FUNCTION "GeneralConditions" : VOID
TITLE =General conditions
VERSION : 0.1

BEGIN
NETWORK
TITLE =Set memoria sempre a "0"
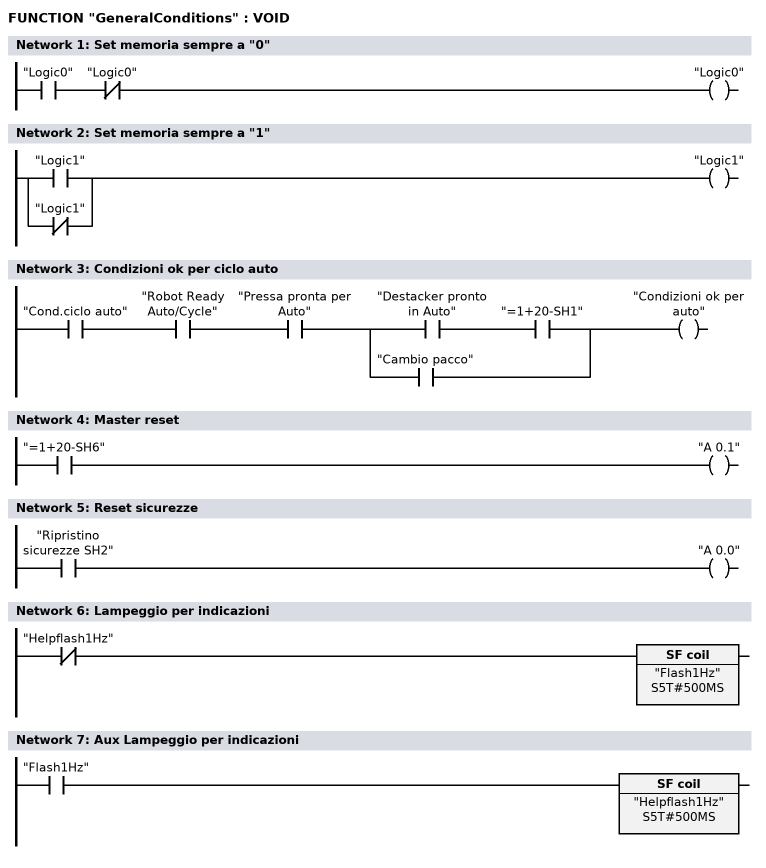
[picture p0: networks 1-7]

      U     "Logic0";
      UN    "Logic0";
      =     "Logic0";
NETWORK
TITLE =Set memoria sempre a "1"

      O     "Logic1";
      ON    "Logic1";
      =     "Logic1";
NETWORK
TITLE =Condizioni ok per ciclo auto

      U     "Cond.ciclo auto";
      U     "Robot Ready Auto/Cycle";
      U     "Pressa pronta per Auto";
      U(    ;
      U     "Destacker pronto in Auto";
      U     "=1+20-SH1";
      O     "Cambio pacco";
      )     ;
      =     "Condizioni ok per auto";
NETWORK
TITLE =Master reset

      U     "=1+20-SH6";
      =     "A 0.1";
NETWORK
TITLE =Reset sicurezze

      U     "Ripristino sicurezze SH2";
      =     "A 0.0";
NETWORK
TITLE =Lampeggio per indicazioni

      UN    "Helpflash1Hz";
      L     S5T#500MS;
      SA    "Flash1Hz";
      NOP   0;
      NOP   0;
      NOP   0;
      NOP   0;
NETWORK
TITLE =Aux Lampeggio per indicazioni

      U     "Flash1Hz";
      L     S5T#500MS;
      SA    "Helpflash1Hz";
      NOP   0;
      NOP   0;
      NOP   0;
      NOP   0;
END_FUNCTION

